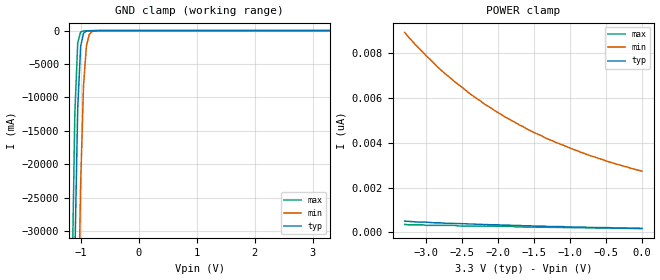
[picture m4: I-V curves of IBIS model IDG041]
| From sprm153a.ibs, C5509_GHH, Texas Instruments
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| Pin_model   IDG041
[Model]   IDG041
 Model_type   Input
 Polarity   Non-Inverting
 Vinl  =  1.08
 Vinh  =  2.1
|Variable   typ   min   max
 C_comp   2.073pF   2.058pF   2.151pF
[Temperature Range]   25   125   -40
[Voltage Range]   3.3   3   3.6
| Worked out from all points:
|   GND clamp passes 1 mA (typ) near -0.60 V on its own axis
[GND Clamp]
|Voltage   I(typ)   I(min)   I(max)
-3.3V     -2.127kA   -2.167kA   -2.109kA
-1.15V    -66.48A    -117.1A    -39.31A
-1.1V     -33.84A    -80.11A    -12.46A
-1.05V    -11.54A    -47.82A    -1.806A
-1V       -2.382A    -22.98A    -205mA
-950mV    -392.1mA   -8.238A    -52.03mA
-900mV    -76.18mA   -2.294A    -31.53mA
-850mV    -25.57mA   -572.4mA   -22.71mA
-800mV    -14.01mA   -143.1mA   -15.62mA
-600mV    -1.042mA   -2.237mA   -712.8uA
3.3V      183pA      3.007nA    153.7pA
[POWER Clamp]
|Voltage   I(typ)   I(min)   I(max)
-3.3V     508pA      8.924nA    361.5pA
-3.15V    472.5pA    8.377nA    342.8pA
-3V       462.7pA    7.88nA     317.1pA
-2.75V    413.9pA    7.115nA    317.1pA
-2.6V     399.7pA    6.714nA    317.1pA
-2.3V     365.9pA    5.977nA    286pA
-1.9V     329.5pA    5.146nA    276.2pA
-1.5V     282.4pA    4.454nA    238.9pA
-1.3V     263.8pA    4.157nA    230.9pA
-950mV    243.4pA    3.701nA    216.7pA
-500mV    217.6pA    3.193nA    196.3pA
0V        183.4pA    2.735nA    171pA
